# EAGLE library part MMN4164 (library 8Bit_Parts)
64Kx1Bit DRAM
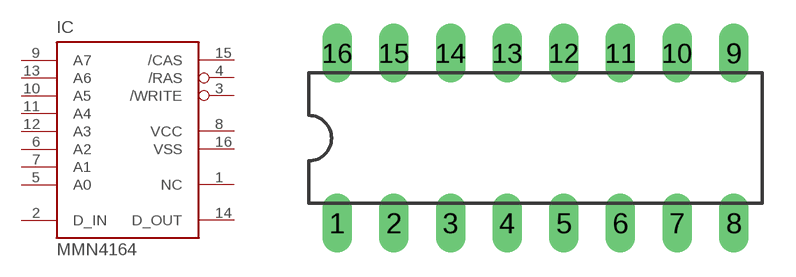
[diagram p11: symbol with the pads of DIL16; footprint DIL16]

Designator prefix IC

## MMN4164  [DIL16]
1  NC  nc
2  D_IN  in
3  /WRITE  in
4  /RAS  in
5  A0  in
6  A2  in
7  A1  in
8  VCC  pwr
9  A7  in
10  A5  in
11  A4  in
12  A3  in
13  A6  in
14  D_OUT  out
15  /CAS  in
16  VSS  pwr

## Footprint DIL16 (pad centres in mm)
Dual In Line Package
drill 0.813 long: 1 -8.89,-3.81; 2 -6.35,-3.81; 3 -3.81,-3.81; 4 -1.27,-3.81; 5 1.27,-3.81; 6 3.81,-3.81; 7 6.35,-3.81; 8 8.89,-3.81; 9 8.89,3.81; 10 6.35,3.81; 11 3.81,3.81; 12 1.27,3.81; 13 -1.27,3.81; 14 -3.81,3.81; 15 -6.35,3.81; 16 -8.89,3.81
